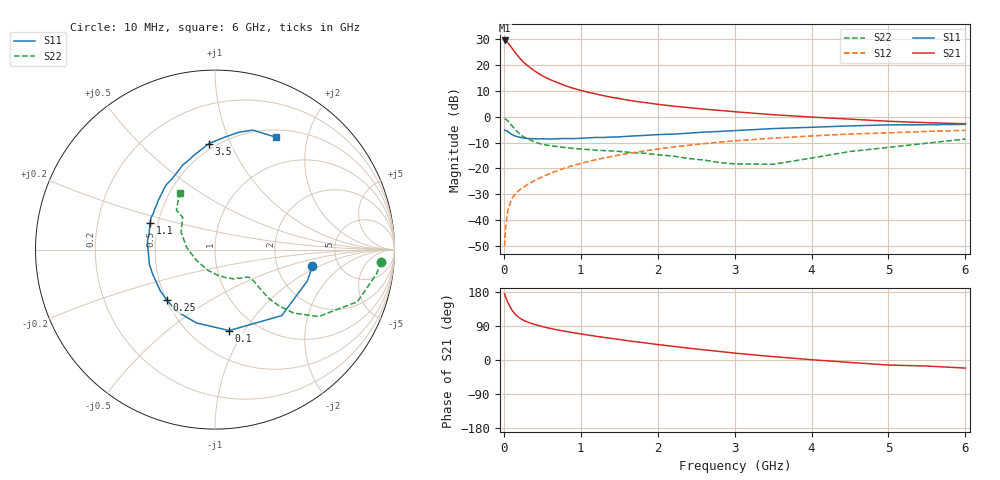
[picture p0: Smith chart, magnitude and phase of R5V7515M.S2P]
! SIEMENS Small Signal Semiconductors
! BFR183
! Si NPN RF Bipolar Junction Transistor in SOT23
! VCE = 0.75 V  IC = 15 mA
! Common Emitter S-Parameters:  May  1996
# GHz  S  MA  R  50
!  f  S11  S21  S12  S22
! GHz  MAG  ANG  MAG  ANG  MAG  ANG  MAG  ANG
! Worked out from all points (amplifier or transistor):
!   36 points, 10 MHz to 6 GHz, reference 50 ohm
!   highest |S21| = 29.6 dB at 10 MHz (marker M1)
!   |S21| within 3 dB of that: start of sweep to 106.5 MHz
!   unconditionally stable (mu >= 1): 466.5 MHz to 3.005 GHz
!   at 250 MHz: K = 0.80, MSG = 24.4 dB, |S12| = -27.4 dB
!   at 1.4 GHz: K = 1.10, MAG = 9.6 dB, |S12| = -15.4 dB
!   at 6 GHz: K = 0.97, MSG = 1.3 dB, |S12| = -5.2 dB
!   S11 on the Smith chart (normalised r, x): 10 MHz: 3.20, -0.85; 100 MHz: 0.75, -0.86; 250 MHz: 0.50, -0.33; 1.1 GHz: 0.45, +0.16; 3.5 GHz: 0.46, +0.83; 6 GHz: 0.60, +1.52
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0.01  0.5509 -9.7  30.27 174.2  0.0031 83.1  0.9279 -4.2
0.02  0.5434 -18.7  29.93 168.3  0.0065 82.1  0.91 -8.6
0.05  0.5231 -44.7  27.7 152.7  0.0149 73.2  0.8449 -20.1
0.1  0.4578 -80.0  22.1 133.2  0.0254 64.7  0.6868 -32.9
0.15  0.4219 -103.8  17.44 120.1  0.0321 60.3  0.5629 -38.9
0.2  0.4051 -121.3  14.13 111.5  0.0377 60.3  0.4748 -41.3
0.25  0.3882 -133.7  11.75 105.3  0.0425 60.4  0.4147 -42.1
0.3  0.382 -142.7  10.05 100.8  0.0478 61.5  0.3772 -41.8
0.4  0.3733 -158.4  7.742 93.8  0.0583 62.9  0.3251 -40.7
0.5  0.3751 -167.4  6.251 88.2  0.0686 64.4  0.2926 -39.6
0.6  0.3708 -175.7  5.286 83.5  0.08 64.9  0.2755 -39.0
0.8  0.3795 172.4  4.019 75.6  0.1022 65.2  0.2532 -39.1
0.9  0.3774 166.7  3.583 72.1  0.1137 64.9  0.2438 -39.3
1.1  0.3913 157.6  2.985 65.6  0.1363 63.8  0.2317 -42.0
1.3  0.3982 149.5  2.564 59.6  0.159 62.1  0.2214 -44.5
1.6  0.4185 139.1  2.122 51.1  0.1925 59.1  0.2069 -50.5
2.2  0.4613 121.2  1.613 36.1  0.2591 51.9  0.1736 -67.0
2.8  0.5205 106.1  1.333 22.6  0.3225 43.9  0.1294 -95.4
3.5  0.5919 93.2  1.099 8.9  0.3857 33.6  0.1199 -150.7
4.5  0.6667 78.6  0.902 -6.5  0.4641 20.0  0.2124 152.8
5.5  0.7025 66.4  0.77 -16.0  0.5217 8.3  0.3079 134.4
6  0.713 61.4  0.734 -21.3  0.5469 0.8  0.371 122.0
